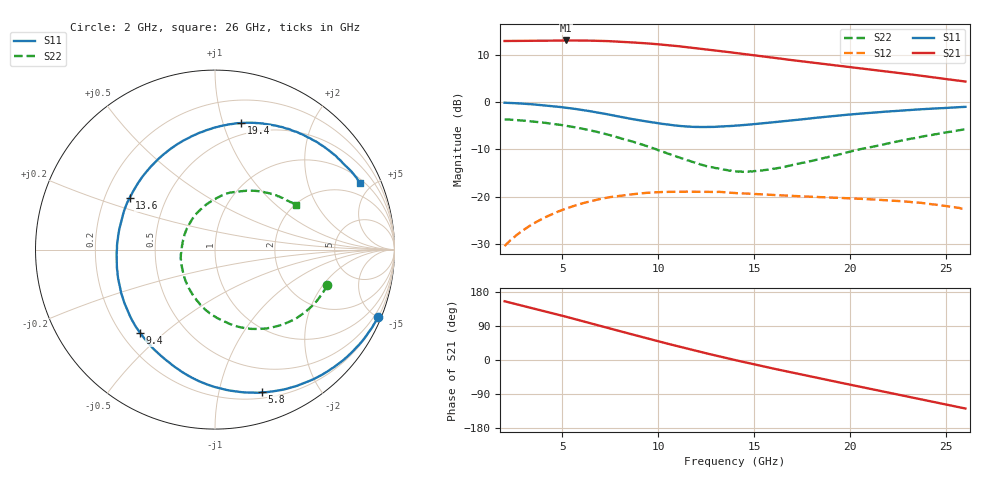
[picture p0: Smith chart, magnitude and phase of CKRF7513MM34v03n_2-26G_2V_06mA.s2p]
! CHUO DENSHI KOGYO Co.,Ltd.
! 22. July 2016
! CKRF7513MM34
! N-channel HJ-FET
! Vds = 2 V Id = 6 mA
# Hz S  MA  R 50
!	f	S11	S21	S12	S22
!	Hz	MAG	ANG	MAG	ANG	MAG	ANG	MAG	ANG
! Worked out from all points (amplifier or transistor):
!   241 points, 2 GHz to 26 GHz, reference 50 ohm
!   highest |S21| = 13.0 dB at 5.2 GHz (marker M1)
!   |S21| within 3 dB of that: start of sweep to 14.75 GHz
!   unconditionally stable (mu >= 1): 14.1 GHz to 21.36 GHz; 21.45504 GHz to 21.53725 GHz
!   at 6 GHz: K = 0.47, MSG = 17.2 dB, |S12| = -21.4 dB
!   at 14 GHz: K = 0.99, MSG = 14.8 dB, |S12| = -19.2 dB
!   at 26 GHz: K = 0.80, MSG = 13.4 dB, |S12| = -22.6 dB
!   lowest NFmin = 0.31 dB at 10 GHz
!   S11 on the Smith chart (normalised r, x): 2 GHz: 0.23, -4.98; 5.8 GHz: 0.25, -1.35; 9.4 GHz: 0.27, -0.42; 13.6 GHz: 0.31, +0.25; 19.4 GHz: 0.39, +1.15; 26 GHz: 1.21, +4.26
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2e9  0.9825 -22.6  4.388 155.0  0.03031 73.0  0.6568 -17.5
3.5e9  0.9433 -40.8  4.416 136.3  0.05224 60.5  0.6222 -31.2
5.2e9  0.8707 -63.2  4.446 114.2  0.07548 45.8  0.5618 -48.0
5.8e9  0.8375 -71.8  4.441 106.2  0.08262 40.4  0.5354 -54.4
6e9  0.8266 -74.6  4.439 103.5  0.08517 38.6  0.5262 -56.6
6.9e9  0.7708 -88.6  4.407 91.3  0.09441 30.6  0.4797 -66.7
7.6e9  0.7252 -100.1  4.357 81.6  0.1002 24.3  0.4399 -75.0
8.6e9  0.6633 -117.1  4.243 68.2  0.1064 16.1  0.3856 -86.9
9.4e9  0.624 -132.0  4.145 57.5  0.1104 9.7  0.3439 -97.8
1e10  0.597 -143.7  4.052 49.5  0.1124 4.9  0.3107 -106.7
1.08e10  0.5684 -159.2  3.912 39.0  0.1134 -1.1  0.2728 -118.7
1.17e10  0.5488 -176.6  3.743 27.6  0.1137 -7.2  0.2368 -134.4
1.27e10  0.5455 164.6  3.545 15.3  0.1129 -13.1  0.2065 -153.2
1.36e10  0.5562 148.8  3.366 4.5  0.1117 -19.2  0.1916 -172.7
1.4e10  0.5621 142.4  3.286 -0.1  0.1101 -21.1  0.1861 179.4
1.61e10  0.6147 113.3  2.907 -23.7  0.1047 -30.5  0.1987 137.9
1.8e10  0.6734 91.9  2.605 -44.0  0.1005 -38.0  0.2398 108.2
1.94e10  0.7197 78.4  2.41 -58.8  0.09792 -43.6  0.2803 90.8
2.06e10  0.756 67.6  2.253 -71.5  0.09536 -48.4  0.3209 77.7
2.2e10  0.7941 56.1  2.081 -86.0  0.09187 -54.4  0.3668 62.9
2.4e10  0.8459 39.6  1.854 -107.2  0.08495 -64.3  0.4415 44.7
2.6e10  0.8889 24.6  1.642 -128.0  0.07425 -74.7  0.5145 28.9
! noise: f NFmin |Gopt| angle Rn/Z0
1e+10  0.31  0.525  97.4  0.08
1.05e+10  0.33  0.509  104.6  0.07
1.1e+10  0.36  0.482  113.1  0.06
1.15e+10  0.37  0.456  123.1  0.05
1.2e+10  0.4  0.439  132.8  0.04
1.25e+10  0.41  0.414  143.3  0.04
1.3e+10  0.44  0.397  155  0.03
1.35e+10  0.48  0.392  166.4  0.03
1.4e+10  0.5  0.392  178.4  0.03
1.5e+10  0.53  0.41  -160.7  0.03
